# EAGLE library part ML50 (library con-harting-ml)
HARTING
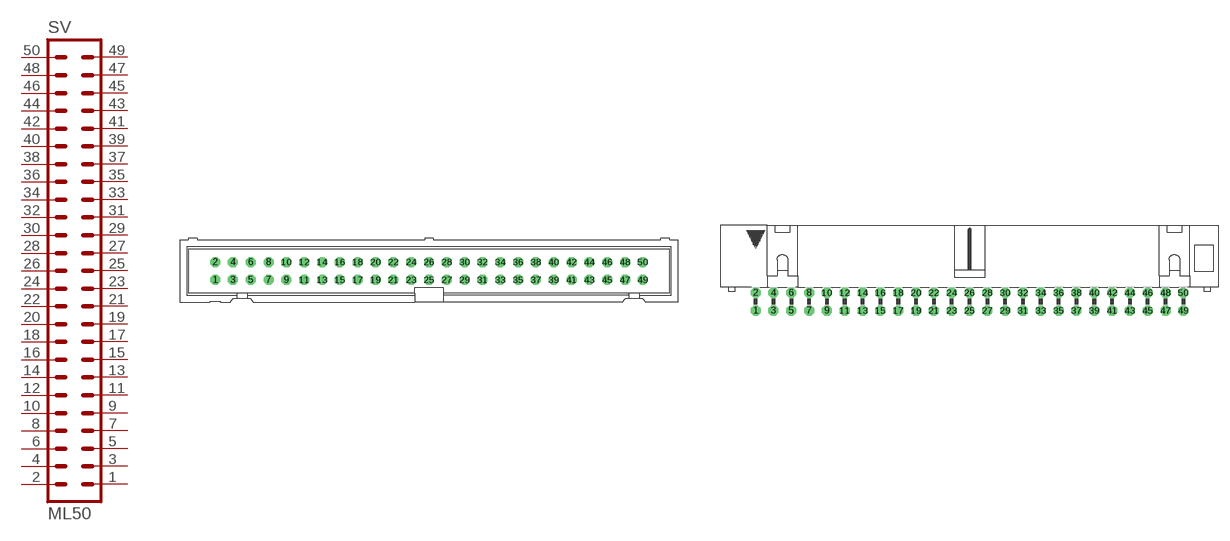
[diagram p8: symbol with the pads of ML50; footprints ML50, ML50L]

Designator prefix SV

## ML50 (OC_FARNELL: unknown; OC_NEWARK: unknown)  [ML50]
1  1  pas
2  2  pas
3  3  pas
4  4  pas
5  5  pas
6  6  pas
7  7  pas
8  8  pas
9  9  pas
10  10  pas
11  11  pas
12  12  pas
13  13  pas
14  14  pas
15  15  pas
16  16  pas
17  17  pas
18  18  pas
19  19  pas
20  20  pas
21  21  pas
22  22  pas
23  23  pas
24  24  pas
25  25  pas
26  26  pas
27  27  pas
28  28  pas
29  29  pas
30  30  pas
31  31  pas
32  32  pas
33  33  pas
34  34  pas
35  35  pas
36  36  pas
37  37  pas
38  38  pas
39  39  pas
40  40  pas
41  41  pas
42  42  pas
43  43  pas
44  44  pas
45  45  pas
46  46  pas
47  47  pas
48  48  pas
49  49  pas
50  50  pas

## ML50L (OC_FARNELL: unknown; OC_NEWARK: unknown)  [ML50L]
Pads as for ML50

## ML503M (OC_FARNELL: unknown; OC_NEWARK: unknown)  [3M_50]
Pads as for ML50

## ML503ML (OC_FARNELL: unknown; OC_NEWARK: unknown)  [3M_50L]
Pads as for ML50

## Footprint ML50 (pad centres in mm)
HARTING
drill 0.914 octagon: 1 -30.48,-1.27; 2 -30.48,1.27; 3 -27.94,-1.27; 4 -27.94,1.27; 5 -25.4,-1.27; 6 -25.4,1.27; 7 -22.86,-1.27; 8 -22.86,1.27; 9 -20.32,-1.27; 10 -20.32,1.27; 11 -17.78,-1.27; 12 -17.78,1.27; 13 -15.24,-1.27; 14 -15.24,1.27; 15 -12.7,-1.27; 16 -12.7,1.27; 17 -10.16,-1.27; 18 -10.16,1.27; 19 -7.62,-1.27; 20 -7.62,1.27; 21 -5.08,-1.27; 22 -5.08,1.27; 23 -2.54,-1.27; 24 -2.54,1.27; 25 0,-1.27; 26 0,1.27; 27 2.54,-1.27; 28 2.54,1.27; 29 5.08,-1.27; 30 5.08,1.27; 31 7.62,-1.27; 32 7.62,1.27; 33 10.16,-1.27; 34 10.16,1.27; 35 12.7,-1.27; 36 12.7,1.27; 37 15.24,-1.27; 38 15.24,1.27; 39 17.78,-1.27; 40 17.78,1.27; 41 20.32,-1.27; 42 20.32,1.27; 43 22.86,-1.27; 44 22.86,1.27; 45 25.4,-1.27; 46 25.4,1.27; 47 27.94,-1.27; 48 27.94,1.27; 49 30.48,-1.27; 50 30.48,1.27

## Footprint ML50L (pad centres in mm)
HARTING
drill 0.914 octagon: 1 -30.48,-1.27; 2 -30.48,1.27; 3 -27.94,-1.27; 4 -27.94,1.27; 5 -25.4,-1.27; 6 -25.4,1.27; 7 -22.86,-1.27; 8 -22.86,1.27; 9 -20.32,-1.27; 10 -20.32,1.27; 11 -17.78,-1.27; 12 -17.78,1.27; 13 -15.24,-1.27; 14 -15.24,1.27; 15 -12.7,-1.27; 16 -12.7,1.27; 17 -10.16,-1.27; 18 -10.16,1.27; 19 -7.62,-1.27; 20 -7.62,1.27; 21 -5.08,-1.27; 22 -5.08,1.27; 23 -2.54,-1.27; 24 -2.54,1.27; 25 0,-1.27; 26 0,1.27; 27 2.54,-1.27; 28 2.54,1.27; 29 5.08,-1.27; 30 5.08,1.27; 31 7.62,-1.27; 32 7.62,1.27; 33 10.16,-1.27; 34 10.16,1.27; 35 12.7,-1.27; 36 12.7,1.27; 37 15.24,-1.27; 38 15.24,1.27; 39 17.78,-1.27; 40 17.78,1.27; 41 20.32,-1.27; 42 20.32,1.27; 43 22.86,-1.27; 44 22.86,1.27; 45 25.4,-1.27; 46 25.4,1.27; 47 27.94,-1.27; 48 27.94,1.27; 49 30.48,-1.27; 50 30.48,1.27

## Footprint 3M_50 (pad centres in mm)
3M
drill 0.813 square: 1 -30.48,-1.27; 2 -30.48,1.27; 3 -27.94,-1.27; 4 -27.94,1.27; 5 -25.4,-1.27; 6 -25.4,1.27; 7 -22.86,-1.27; 8 -22.86,1.27; 9 -20.32,-1.27; 10 -20.32,1.27; 11 -17.78,-1.27; 12 -17.78,1.27; 13 -15.24,-1.27; 14 -15.24,1.27; 15 -12.7,-1.27; 16 -12.7,1.27; 17 -10.16,-1.27; 18 -10.16,1.27; 19 -7.62,-1.27; 20 -7.62,1.27; 21 -5.08,-1.27; 22 -5.08,1.27; 23 -2.54,-1.27; 24 -2.54,1.27; 25 0,-1.27; 26 0,1.27; 27 2.54,-1.27; 28 2.54,1.27; 29 5.08,-1.27; 30 5.08,1.27; 31 7.62,-1.27; 32 7.62,1.27; 33 10.16,-1.27; 34 10.16,1.27; 35 12.7,-1.27; 36 12.7,1.27; 37 15.24,-1.27; 38 15.24,1.27; 39 17.78,-1.27; 40 17.78,1.27; 41 20.32,-1.27; 42 20.32,1.27; 43 22.86,-1.27; 44 22.86,1.27; 45 25.4,-1.27; 46 25.4,1.27; 47 27.94,-1.27; 48 27.94,1.27; 49 30.48,-1.27; 50 30.48,1.27

## Footprint 3M_50L (pad centres in mm)
3M
drill 0.813 square: 1 -30.48,-5.08; 2 -30.48,-2.54; 3 -27.94,-5.08; 4 -27.94,-2.54; 5 -25.4,-5.08; 6 -25.4,-2.54; 7 -22.86,-5.08; 8 -22.86,-2.54; 9 -20.32,-5.08; 10 -20.32,-2.54; 11 -17.78,-5.08; 12 -17.78,-2.54; 13 -15.24,-5.08; 14 -15.24,-2.54; 15 -12.7,-5.08; 16 -12.7,-2.54; 17 -10.16,-5.08; 18 -10.16,-2.54; 19 -7.62,-5.08; 20 -7.62,-2.54; 21 -5.08,-5.08; 22 -5.08,-2.54; 23 -2.54,-5.08; 24 -2.54,-2.54; 25 0,-5.08; 26 0,-2.54; 27 2.54,-5.08; 28 2.54,-2.54; 29 5.08,-5.08; 30 5.08,-2.54; 31 7.62,-5.08; 32 7.62,-2.54; 33 10.16,-5.08; 34 10.16,-2.54; 35 12.7,-5.08; 36 12.7,-2.54; 37 15.24,-5.08; 38 15.24,-2.54; 39 17.78,-5.08; 40 17.78,-2.54; 41 20.32,-5.08; 42 20.32,-2.54; 43 22.86,-5.08; 44 22.86,-2.54; 45 25.4,-5.08; 46 25.4,-2.54; 47 27.94,-5.08; 48 27.94,-2.54; 49 30.48,-5.08; 50 30.48,-2.54
hole 2.54 at -36.398,-3.277
hole 2.54 at 36.398,-3.277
